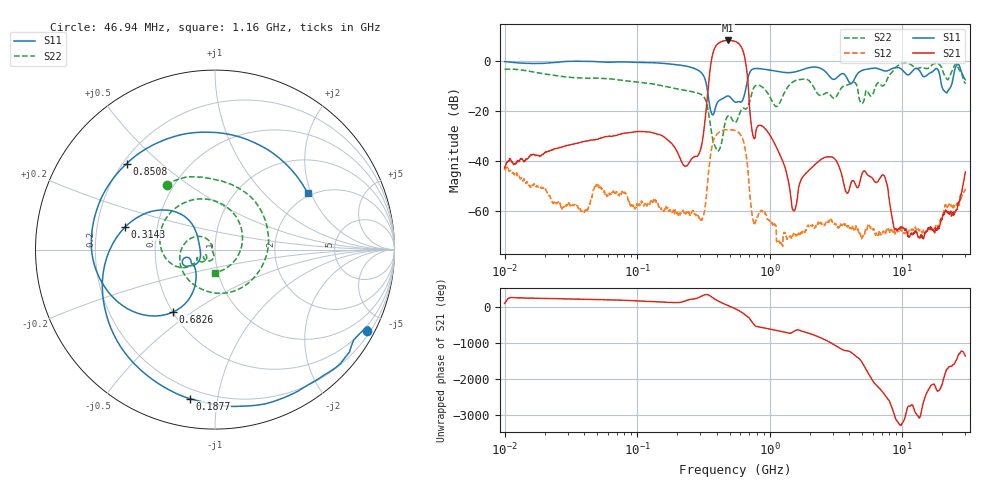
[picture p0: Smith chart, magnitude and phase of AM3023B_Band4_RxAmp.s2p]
# Hz S DB R 50.0
!freq dBS11 angS11 dBS21 angS21 dBS12 angS12 dBS22 angS22
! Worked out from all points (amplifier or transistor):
!   1601 points, 10 MHz to 30 GHz, reference 50 ohm
!   highest |S21| = 8.0 dB at 483.3 MHz (marker M1)
!   |S21| within 3 dB of that: 385.4 MHz to 616.7 MHz (231.3 MHz wide, 46.2 % of centre)
!   unconditionally stable (mu >= 1): start of sweep to end of sweep
!   at 37.85 MHz: K = 1071.78, MAG = -19.5 dB, |S12| = -60.1 dB
!   at 547.7 MHz: K = 5.03, MAG = 7.8 dB, |S12| = -27.8 dB
!   at 30 GHz: K = 21971.17, MAG = -43.1 dB, |S12| = -51.1 dB
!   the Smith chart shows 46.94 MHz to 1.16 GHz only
!   S11 on the Smith chart (normalised r, x): 46.94 MHz: 0.35, -3.97; 187.7 MHz: 0.15, -0.83; 314.3 MHz: 0.32, +0.11; 682.6 MHz: 0.50, -0.42; 850.8 MHz: 0.21, +0.39; 1.16 GHz: 1.91, +1.89
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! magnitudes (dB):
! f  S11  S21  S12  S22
! 10 MHz  -0.4  -42.8  -43.8  -3.5
! 38.04 MHz  -0.3  -32.5  -60.0  -7.0
! 46.94 MHz  -0.4  -31.6  -51.6  -7.0
! 144.7 MHz  -1.0  -29.4  -58.3  -9.8
! 187.7 MHz  -1.5  -33.9  -59.7  -11.0
! 233.9 MHz  -2.2  -42.1  -61.2  -11.9
! 314.3 MHz  -5.7  -30.5  -62.4  -14.1
! 374.5 MHz  -21.7  3.2  -32.4  -32.1
! 483.3 MHz  -14.1  8.0  -27.6  -22.1
! 547.7 MHz  -16.6  7.7  -27.8  -24.7
! 682.6 MHz  -7.5  -7.4  -42.5  -18.5
! 750.7 MHz  -3.3  -30.2  -63.8  -11.4
! 850.8 MHz  -3.3  -25.8  -60.9  -10.1
! 1.16 GHz  -4.4  -36.1  -72.4  -17.9
! 1.52 GHz  -4.6  -60.0  -69.0  -8.3
! 2.084 GHz  -2.6  -42.7  -65.9  -9.5
! 4.977 GHz  -4.0  -45.2  -70.6  -17.1
! 7.926 GHz  -3.9  -54.1  -67.4  -6.2
! 8.893 GHz  -2.8  -67.2  -69.1  -3.0
! 14.09 GHz  -5.7  -69.8  -68.7  -2.7
! 25.05 GHz  -3.3  -60.4  -58.4  -1.6
! 30 GHz  -7.7  -44.4  -51.1  -9.3
